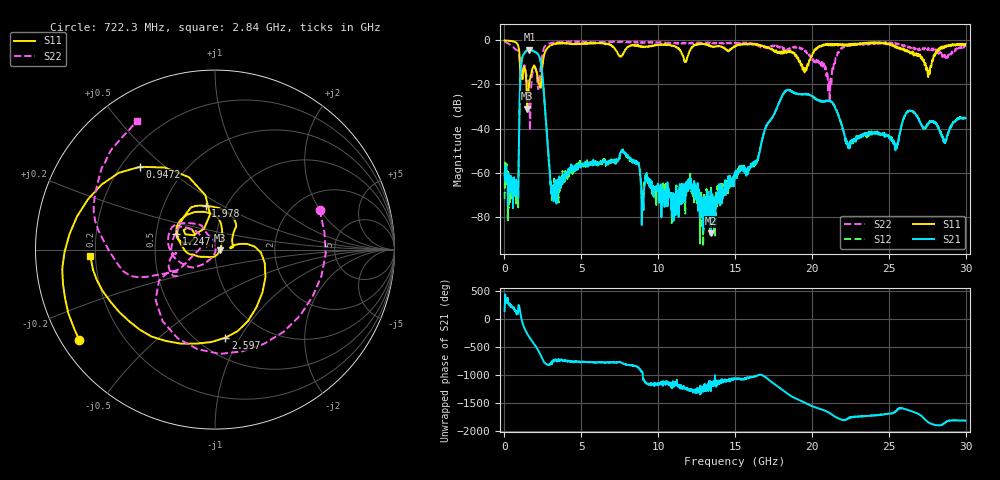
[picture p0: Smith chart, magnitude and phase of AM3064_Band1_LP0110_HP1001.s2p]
# Hz S DB R 50.0
!freq dBS11 angS11 dBS21 angS21 dBS12 angS12 dBS22 angS22
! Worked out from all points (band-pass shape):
!   1600 points, 10 MHz to 29.98 GHz, reference 50 ohm
!   highest |S21| = -4.29 dB at 1.622 GHz (marker M1); lowest = -87.5 dB at 13.43 GHz (marker M2)
!   |S21| within 3 dB of the highest: 1.183 GHz to 2.257 GHz (1.074 GHz wide, 62.4 % of centre)
!   lowest |S11| = -30.9 dB at 1.472 GHz (marker M3), VSWR 1.06, Z = 52.9 - j0.362 ohm
!   |S11| at or under -10 dB: 1.002 GHz to 2.501 GHz (1.499 GHz wide, 85.6 % of centre); 19.24 GHz to 19.8 GHz (559.9 MHz wide, 2.87 % of centre); 27.3 GHz to 27.8 GHz (498.2 MHz wide, 1.81 % of centre)
!   |S22| runs from -40.8 to -0.4 dB; largest |S21 - S12| = 0.008
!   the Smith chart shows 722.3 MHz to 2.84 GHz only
!   S11 on the Smith chart (normalised r, x): 722.3 MHz: 0.05, -0.30; 947.2 MHz: 0.28, +0.41; 1.247 GHz: 0.64, +0.12; 1.978 GHz: 0.80, +0.42; 2.597 GHz: 0.67, -0.87; 2.84 GHz: 0.18, -0.03
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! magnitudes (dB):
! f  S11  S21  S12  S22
! 10 MHz  0.0  -60.2  -72.0  -0.4
! 722.3 MHz  -0.8  -69.8  -64.1  -4.1
! 947.2 MHz  -4.1  -43.6  -43.4  -6.1
! 1.247 GHz  -12.6  -6.3  -6.3  -11.8
! 1.472 GHz  -30.9  -4.5  -4.5  -16.8
! 1.622 GHz  -19.0  -4.3  -4.2  -26.9
! 1.978 GHz  -12.1  -5.2  -5.2  -12.4
! 2.597 GHz  -6.1  -27.1  -26.9  -3.0
! 2.84 GHz  -3.2  -49.4  -49.4  -1.5
! 3.271 GHz  -1.6  -64.8  -65.6  -0.9
! 5.015 GHz  -1.6  -57.2  -56.5  -0.7
! 7.714 GHz  -6.2  -50.4  -49.9  -0.7
! 10 GHz  -2.0  -67.6  -66.8  -0.9
! 13.43 GHz  -2.8  -87.5  -66.8  -1.3
! 15 GHz  -2.8  -61.1  -61.2  -1.3
! 18.25 GHz  -5.1  -23.2  -23.2  -4.4
! 19.99 GHz  -7.2  -25.3  -25.2  -8.1
! 21.15 GHz  -1.8  -27.4  -27.6  -27.7
! 22.37 GHz  -2.3  -47.6  -47.9  -2.0
! 25 GHz  -1.4  -43.4  -43.5  -1.3
! 27.56 GHz  -16.6  -38.0  -37.7  -3.6
! 29.98 GHz  -1.6  -35.4  -35.2  -2.8
